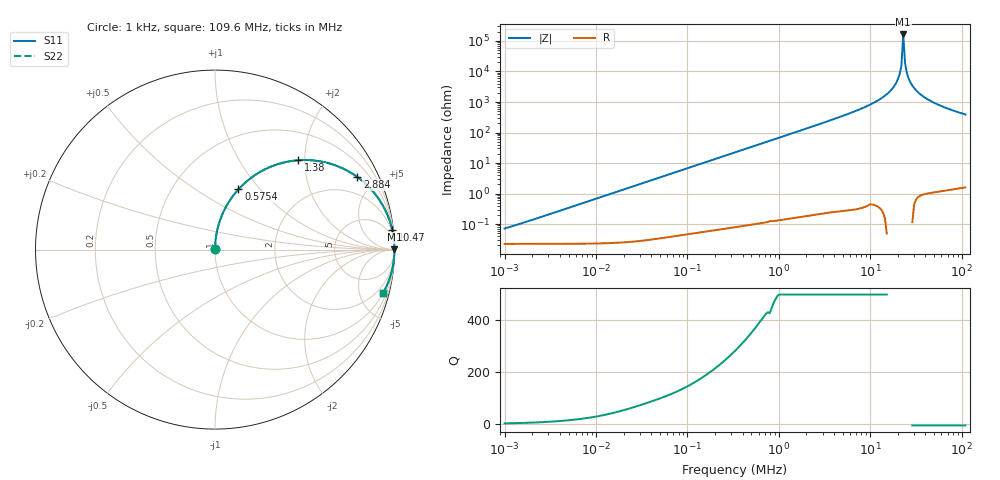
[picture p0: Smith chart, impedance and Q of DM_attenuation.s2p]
! EM Consulting and Software
! Touchstone file was created on 2026-03-09  16:25:53
# HZ S RI R 50.0000
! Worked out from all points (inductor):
!   253 points, 1 kHz to 109.6 MHz, reference 50 ohm
!   read as one part in series: L = 10.8 uH near 1.047 kHz
!   highest |Z| = 163 kohm at 22.91 MHz (marker M1)
!   self-resonance near 22.91 MHz
!   S11 on the Smith chart (normalised r, x): 1 kHz: 1.00, +0.00; 575.4 kHz: 1.00, +0.77; 1.38 MHz: 1.00, +1.86; 2.884 MHz: 1.00, +3.93; 10.47 MHz: 1, +18; 109.6 MHz: 1.03, -7.80
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1000  0.000224 0.000676  0.9998 -0.000676  0.9998 -0.000676  0.000224 0.000676
6918.31  0.000249 0.00468  0.9998 -0.00468  0.9998 -0.00468  0.000249 0.00468
47863.01  0.00137 0.0322  0.9986 -0.0322  0.9986 -0.0322  0.00137 0.0322
331131.1  0.0478 0.2115  0.9522 -0.2115  0.9522 -0.2115  0.0478 0.2115
575439.9  0.1304 0.3355  0.8696 -0.3355  0.8696 -0.3355  0.1304 0.3355
1380384  0.4629 0.4978  0.5371 -0.4978  0.5371 -0.4978  0.4629 0.4978
2290868  0.7058 0.455  0.2942 -0.455  0.2942 -0.455  0.7058 0.455
2884032  0.7936 0.4041  0.2064 -0.4041  0.2064 -0.4041  0.7936 0.4041
5011872  0.9253 0.2625  0.0747 -0.2625  0.0747 -0.2625  0.9253 0.2625
1.047129e7  0.9874 0.1115  0.0126 -0.1115  0.0126 -0.1115  0.9874 0.1115
1.659587e7  0.9982 0.0429  0.00184 -0.0429  0.00184 -0.0429  0.9982 0.0429
1.905461e7  0.9994 0.0245  0.000589 -0.0245  0.000589 -0.0245  0.9994 0.0245
2.089296e7  0.9999 0.0125  0.000143 -0.0125  0.000143 -0.0125  0.9999 0.0125
2.187762e7  1 0.00654  3.01e-05 -0.00654  3.01e-05 -0.00654  1 0.00654
2.290868e7  1 0.000612  -1.15e-05 -0.000612  -1.15e-05 -0.000612  1 0.000612
2.398833e7  1 -0.00531  1.77e-05 0.00531  1.77e-05 0.00531  1 -0.00531
2.511886e7  0.9999 -0.0112  0.000117 0.0112  0.000117 0.0112  0.9999 -0.0112
2.754229e7  0.9995 -0.0231  0.000531 0.0231  0.000531 0.0231  0.9995 -0.0231
3.019952e7  0.9988 -0.0351  0.00124 0.0351  0.00124 0.0351  0.9988 -0.0351
3.630781e7  0.9964 -0.0596  0.0036 0.0596  0.0036 0.0596  0.9964 -0.0596
4.786301e7  0.99 -0.0988  0.00997 0.0988  0.00997 0.0988  0.99 -0.0988
1.096478e8  0.9374 -0.2402  0.0626 0.2402  0.0626 0.2402  0.9374 -0.2402
